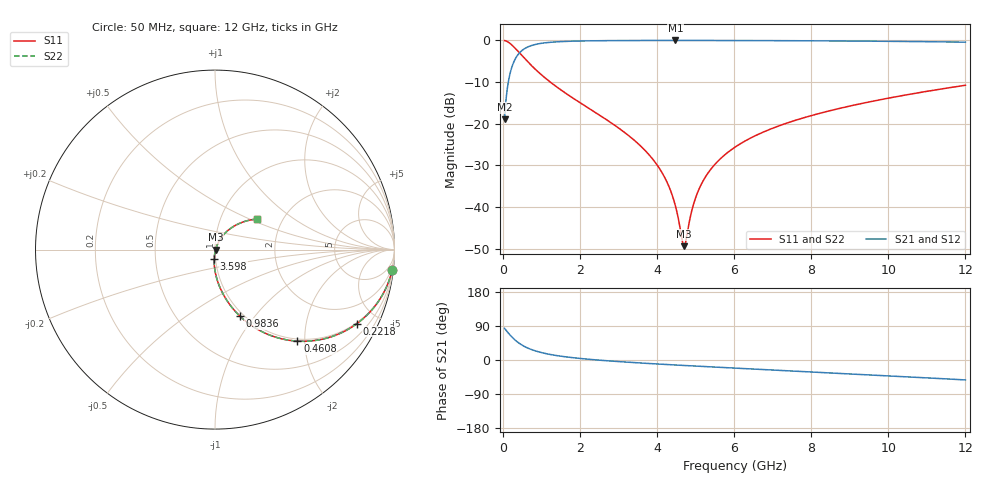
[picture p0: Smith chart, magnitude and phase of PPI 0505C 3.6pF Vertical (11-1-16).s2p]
# GHz S MA R 50
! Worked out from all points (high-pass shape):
!   1601 points, 50 MHz to 12 GHz, reference 50 ohm
!   highest |S21| = -0.03 dB at 4.479 GHz (marker M1); lowest = -18.9 dB at 50 MHz (marker M2)
!   |S21| within 3 dB of the highest: 434.4 MHz to end of sweep
!   lowest |S11| = -49.4 dB at 4.703 GHz (marker M3), VSWR 1.01, Z = 50.3 - j0.0938 ohm
!   |S11| at or under -10 dB: 1.232 GHz to end of sweep
!   |S22| runs from -49.4 to -0.1 dB; largest |S21 - S12| = 0
!   S11 on the Smith chart (normalised r, x): 50 MHz: 1, -17; 221.8 MHz: 0.96, -3.86; 460.8 MHz: 0.96, -1.85; 983.6 MHz: 0.96, -0.84; 3.598 GHz: 0.99, -0.10; 12 GHz: 1.49, +0.55
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0.05  0.9936 -6.6  0.1131 83.3  0.1131 83.3  0.9936 -6.6
0.1470937  0.9481 -19.0  0.3177 71.0  0.3177 71.0  0.9481 -19.0
0.2217813  0.8921 -27.5  0.4512 62.5  0.4512 62.5  0.8921 -27.5
0.4607812  0.6864 -48.0  0.7262 41.9  0.7262 41.9  0.6864 -48.0
0.6923125  0.5275 -60.2  0.8482 29.7  0.8482 29.7  0.5275 -60.2
0.9835938  0.3933 -69.6  0.9177 20.1  0.9177 20.1  0.3933 -69.6
2.044156  0.1737 -85.6  0.9824 3.7  0.9824 3.7  0.1737 -85.6
3.597656  0.05274 -94.8  0.9954 -8.1  0.9954 -8.1  0.05274 -94.8
4.038312  0.03025 -94.8  0.9962 -10.7  0.9962 -10.7  0.03025 -94.8
4.29225  0.01844 -92.1  0.9963 -12.1  0.9963 -12.1  0.01844 -92.1
4.478969  0.01032 -84.6  0.9964 -13.2  0.9964 -13.2  0.01032 -84.6
4.65075  0.004081 -48.8  0.9963 -14.1  0.9963 -14.1  0.004081 -48.8
4.703031  0.003376 -16.0  0.9963 -14.4  0.9963 -14.4  0.003376 -16.0
4.755312  0.003999 17.2  0.9963 -14.7  0.9963 -14.7  0.003999 17.2
4.964437  0.01134 56.3  0.9962 -15.8  0.9962 -15.8  0.01134 56.3
5.181031  0.01986 62.7  0.9959 -17.0  0.9959 -17.0  0.01986 62.7
5.532063  0.03349 64.9  0.9954 -18.8  0.9954 -18.8  0.03349 64.9
6.025  0.05212 64.4  0.9944 -21.4  0.9944 -21.4  0.05212 64.4
6.8615  0.08289 61.5  0.992 -25.7  0.992 -25.7  0.08289 61.5
8.019156  0.1253 56.4  0.987 -31.5  0.987 -31.5  0.1253 56.4
10.01331  0.2026 46.6  0.9732 -41.8  0.9732 -41.8  0.2026 46.6
12  0.2888 36.2  0.9503 -52.6  0.9503 -52.6  0.2888 36.2
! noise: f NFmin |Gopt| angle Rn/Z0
0.05  0.0006498  0.9268  1.823  0.001969
1.372  0.005237  0.7423  4.995  0.004069
2.701  0.008466  0.6949  8.757  0.005385
4.031  0.01135  0.667  12.54  0.006463
5.36  0.01407  0.6486  16.28  0.007455
6.682  0.01673  0.6365  19.93  0.008426
8.012  0.01942  0.6291  23.53  0.009434
9.341  0.02218  0.6255  27.05  0.01051
10.67  0.02506  0.6253  30.5  0.0117
12  0.02812  0.6281  33.88  0.01303
